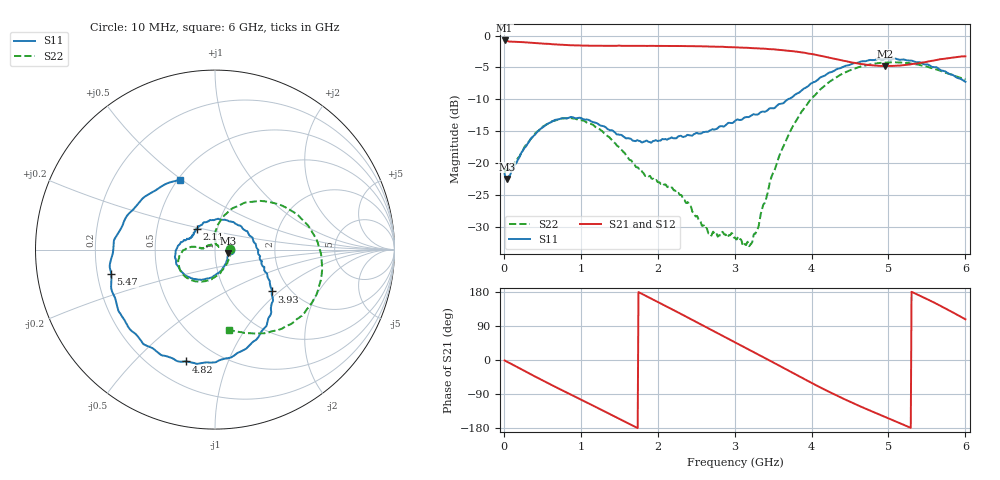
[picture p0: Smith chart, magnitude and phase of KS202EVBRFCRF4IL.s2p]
!Agilent Technologies,N5230A,MY45001650,A.07.50.48
!Agilent N5230A: A.07.50.48
!Date: Monday, June 12, 2017 12:54:31
!Correction: S11(Full 2 Port(1,2))
!S21(Full 2 Port(1,2))
!S12(Full 2 Port(1,2))
!S22(Full 2 Port(1,2))
!S2P File: Measurements: S11, S21, S12, S22:
# Hz S  dB  R 50
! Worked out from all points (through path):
!   600 points, 10 MHz to 6 GHz, reference 50 ohm
!   highest |S21| = -0.77 dB at 10 MHz (marker M1); lowest = -4.8 dB at 4.96 GHz (marker M2)
!   group delay of S21, straight-line fit = 285 ps
!   lowest |S11| = -22.5 dB at 40 MHz (marker M3), VSWR 1.16, Z = 57.7 - j2.43 ohm
!   |S11| at or under -10 dB: start of sweep to 3.688 GHz
!   |S22| runs from -33.0 to -4.2 dB; largest |S21 - S12| = 0.0025
!   S11 on the Smith chart (normalised r, x): 10 MHz: 1.18, -0.00; 2.11 GHz: 0.80, +0.19; 3.93 GHz: 1.62, -0.89; 4.82 GHz: 0.34, -0.72; 5.47 GHz: 0.26, -0.11; 6 GHz: 0.51, +0.49
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1e7  -21.67 -0.4  -0.77 -1.2  -0.77 -1.2  -21.50 0.7
4e7  -22.46 -16.2  -0.85 -4.3  -0.85 -4.3  -20.95 -13.3
2.8e8  -17.48 -84.0  -1.06 -30.1  -1.06 -30.1  -17.27 -79.6
5.5e8  -13.96 -124.8  -1.29 -58.6  -1.29 -58.6  -13.95 -117.1
1.01e9  -12.96 -171.4  -1.56 -105.4  -1.56 -105.2  -13.28 -160.1
1.53e9  -15.58 159.1  -1.61 -158.1  -1.61 -157.9  -17.90 173.0
1.77e9  -16.53 152.3  -1.61 177.2  -1.61 177.3  -20.82 172.8
2.01e9  -16.50 139.2  -1.62 152.2  -1.62 152.4  -22.99 175.5
2.11e9  -16.26 131.5  -1.63 141.8  -1.63 141.9  -23.40 174.1
2.56e9  -15.34 76.5  -1.68 94.3  -1.68 94.4  -29.22 125.5
3.01e9  -13.32 18.9  -1.84 46.4  -1.84 46.5  -31.70 34.4
3.21e9  -12.57 1.3  -1.95 25.0  -1.95 25.1  -32.64 58.5
3.47e9  -11.38 -13.8  -2.13 -3.0  -2.13 -2.8  -22.46 89.8
3.93e9  -8.13 -36.4  -2.75 -52.9  -2.74 -53.0  -11.02 61.3
4.01e9  -7.38 -40.9  -2.91 -61.4  -2.92 -61.4  -9.74 54.5
4.34e9  -5.21 -64.7  -3.75 -95.1  -3.75 -95.1  -6.41 26.9
4.82e9  -3.83 -104.4  -4.69 -138.5  -4.69 -138.6  -4.41 -8.0
4.96e9  -3.64 -116.1  -4.78 -150.4  -4.78 -150.5  -4.24 -17.3
5.01e9  -3.69 -120.1  -4.76 -154.7  -4.76 -154.8  -4.21 -20.6
5.47e9  -4.52 -166.9  -4.18 163.7  -4.18 163.7  -4.77 -49.5
5.73e9  -5.58 159.3  -3.63 137.1  -3.63 137.1  -5.77 -65.0
6e9  -7.24 116.6  -3.25 107.3  -3.26 107.2  -6.88 -80.0
